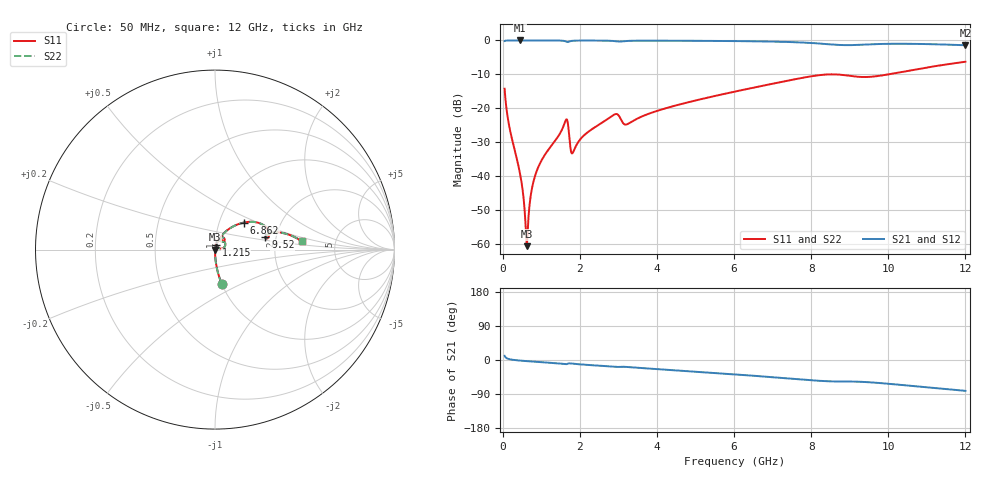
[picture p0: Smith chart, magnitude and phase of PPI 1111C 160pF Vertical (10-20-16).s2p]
# GHz S MA R 50
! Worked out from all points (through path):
!   1601 points, 50 MHz to 12 GHz, reference 50 ohm
!   highest |S21| = -0.01 dB at 445.8 MHz (marker M1); lowest = -1.4 dB at 12 GHz (marker M2)
!   group delay of S21, straight-line fit = 18.6 ps
!   lowest |S11| = -60.8 dB at 625.1 MHz (marker M3), VSWR 1.00, Z = 50.1 - j0.00254 ohm
!   |S11| at or under -10 dB: start of sweep to 10.01 GHz
!   |S22| runs from -60.8 to -6.3 dB; largest |S21 - S12| = 0
!   S11 on the Smith chart (normalised r, x): 50 MHz: 1.00, -0.39; 1.215 GHz: 1.01, +0.05; 6.862 GHz: 1.31, +0.42; 9.52 GHz: 1.75, +0.27; 12 GHz: 2.83, +0.35
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0.05  0.1934 -79.0  0.9808 10.9  0.9808 10.9  0.1934 -79.0
0.1844375  0.04911 -87.4  0.9982 1.9  0.9982 1.9  0.04911 -87.4
0.4458437  0.01105 -87.4  0.9991 -1.5  0.9991 -1.5  0.01105 -87.4
0.5205313  0.005964 -84.1  0.9991 -2.1  0.9991 -2.1  0.005964 -84.1
0.58775  0.002162 -68.4  0.9991 -2.7  0.9991 -2.7  0.002162 -68.4
0.6250938  0.0009145 -1.6  0.999 -3.0  0.999 -3.0  0.0009145 -1.6
0.6624375  0.002129 60.5  0.999 -3.3  0.999 -3.3  0.002129 60.5
0.7520625  0.0062 76.7  0.9989 -3.9  0.9989 -3.9  0.0062 76.7
0.8342188  0.00976 79.2  0.9988 -4.5  0.9988 -4.5  0.00976 79.2
1.215125  0.02565 79.2  0.998 -7.2  0.998 -7.2  0.02565 79.2
1.633375  0.0658 52.5  0.9689 -11.1  0.9689 -11.1  0.0658 52.5
1.805156  0.02145 43.2  0.9867 -9.5  0.9867 -9.5  0.02145 43.2
2.044156  0.03638 72.1  0.9953 -11.7  0.9953 -11.7  0.03638 72.1
2.903062  0.08087 57.9  0.9773 -18.2  0.9773 -18.2  0.08087 57.9
3.209281  0.05738 54.4  0.9812 -18.3  0.9812 -18.3  0.05738 54.4
4.038312  0.09234 63.2  0.9914 -24.2  0.9914 -24.2  0.09234 63.2
6.025  0.1756 50.1  0.9783 -38.0  0.9783 -38.0  0.1756 50.1
6.8615  0.2211 43.0  0.9646 -44.3  0.9646 -44.3  0.2211 43.0
8.019156  0.2963 28.7  0.9154 -53.6  0.9154 -53.6  0.2963 28.7
9.520375  0.2898 14.2  0.8755 -58.8  0.8755 -58.8  0.2898 14.2
10.01331  0.3161 16.5  0.8913 -62.8  0.8913 -62.8  0.3161 16.5
12  0.4846 5.6  0.8492 -81.4  0.8492 -81.4  0.4846 5.6
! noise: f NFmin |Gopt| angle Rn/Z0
0.05  0.0003925  0.8726  0.3428  0.000664
1.372  0.005559  0.7675  6.439  0.004851
2.701  0.0127  0.7977  12.65  0.01284
4.031  0.01251  0.7118  18.59  0.008336
5.36  0.01497  0.6894  24.34  0.008974
6.682  0.02337  0.7484  30.24  0.01745
8.012  0.05456  0.8653  36.28  0.07861
9.341  0.09275  0.908  41.9  0.1931
10.67  0.0621  0.8521  47.01  0.07539
12  0.05314  0.8157  51.75  0.04892
